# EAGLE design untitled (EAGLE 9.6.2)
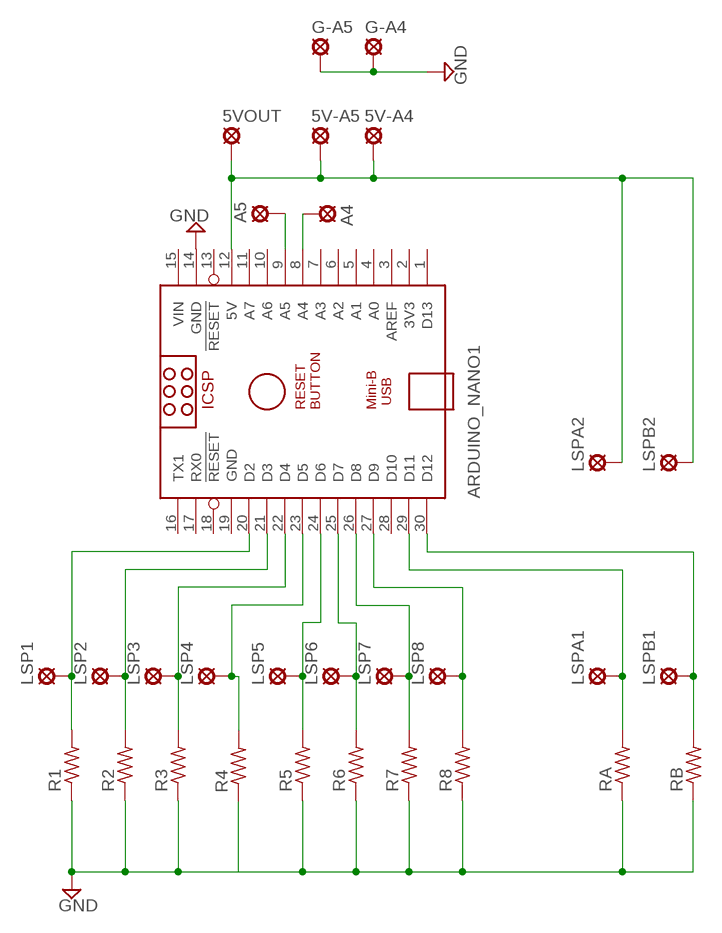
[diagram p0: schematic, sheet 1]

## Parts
5V-A4  LSP10  [LSP10]
5V-A5  LSP10  [LSP10]
5VOUT  LSP10  [LSP10]
A4  LSP10  [LSP10]
A5  LSP10  [LSP10]
ARDUINO_NANO1  ARDUINO_NANO  [ARDUINO_NANO]
G-A4  LSP10  [LSP10]
G-A5  LSP10  [LSP10]
LSP1  LSP10  [LSP10]
LSP2  LSP10  [LSP10]
LSP3  LSP10  [LSP10]
LSP4  LSP10  [LSP10]
LSP5  LSP10  [LSP10]
LSP6  LSP10  [LSP10]
LSP7  LSP10  [LSP10]
LSP8  LSP10  [LSP10]
LSPA1  LSP10  [LSP10]
LSPA2  LSP10  [LSP10]
LSPB1  LSP10  [LSP10]
LSPB2  LSP10  [LSP10]
R1  R-US_0309/12  [0309/12]
R2  R-US_0309/12  [0309/12]
R3  R-US_0309/12  [0309/12]
R4  R-US_0309/12  [0309/12]
R5  R-US_0309/12  [0309/12]
R6  R-US_0309/12  [0309/12]
R7  R-US_0309/12  [0309/12]
R8  R-US_0309/12  [0309/12]
RA  R-US_0309/12  [0309/12]
RB  R-US_0309/12  [0309/12]

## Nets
GND: ARDUINO_NANO1.14(GND) G-A4.MP G-A5.MP R1.1 R2.1 R3.1 R4.1 R5.1 R6.1 R7.1 R8.1 RA.1 RB.1
N$1: 5V-A4.MP 5V-A5.MP 5VOUT.MP ARDUINO_NANO1.12(5V) LSPA2.MP LSPB2.MP
N$2: ARDUINO_NANO1.20(D2) LSP1.MP R1.2
N$3: A5.MP ARDUINO_NANO1.9(A5)
N$4: ARDUINO_NANO1.21(D3) LSP2.MP R2.2
N$5: ARDUINO_NANO1.22(D4) LSP3.MP R3.2
N$6: ARDUINO_NANO1.23(D5) LSP4.MP R4.2
N$7: ARDUINO_NANO1.24(D6) LSP5.MP R5.2
N$8: ARDUINO_NANO1.25(D7) LSP6.MP R6.2
N$9: ARDUINO_NANO1.26(D8) LSP7.MP R7.2
N$10: ARDUINO_NANO1.27(D9) LSP8.MP R8.2
N$11: ARDUINO_NANO1.30(D12) LSPB1.MP RB.2
N$12: ARDUINO_NANO1.29(D11) LSPA1.MP RA.2
N$13: A4.MP ARDUINO_NANO1.8(A4)
Unconnected: ARDUINO_NANO1.1(D13) ARDUINO_NANO1.2(3V3) ARDUINO_NANO1.3(AREF) ARDUINO_NANO1.4(A0) ARDUINO_NANO1.5(A1) ARDUINO_NANO1.6(A2) ARDUINO_NANO1.7(A3) ARDUINO_NANO1.10(A6) ARDUINO_NANO1.11(A7) ARDUINO_NANO1.13(!RESET) ARDUINO_NANO1.16(TX1) ARDUINO_NANO1.17(RX0) ARDUINO_NANO1.18(!RESET) ARDUINO_NANO1.28(D10)

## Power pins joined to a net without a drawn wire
GND: ARDUINO_NANO1.19(GND)
VIN: ARDUINO_NANO1.15(VIN)

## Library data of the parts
5V-A4 5V-A5 5VOUT A4 A5 G-A4 G-A5 LSP1-LSP8 LSPA1 LSPA2 LSPB1 LSPB2 = solpad:LSP10: SOLDER PAD
ARDUINO_NANO1 = ArduinoNanoV30:ARDUINO_NANO: Arduino Nano V3.0 Overview: The Arduino Nano is a small, complete, and breadboard-friendly board based on the ATmega328 (Arduino Nano 3.x) or ATmega168 (Arduino Nano 2.x). It has more or less the same functionality of the Arduino Duemilanove, but in a different package. It lacks only a DC power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
R1-R8 RA RB = rcl:R-US_: RESISTOR, American symbol; SPICEPREFIX: R

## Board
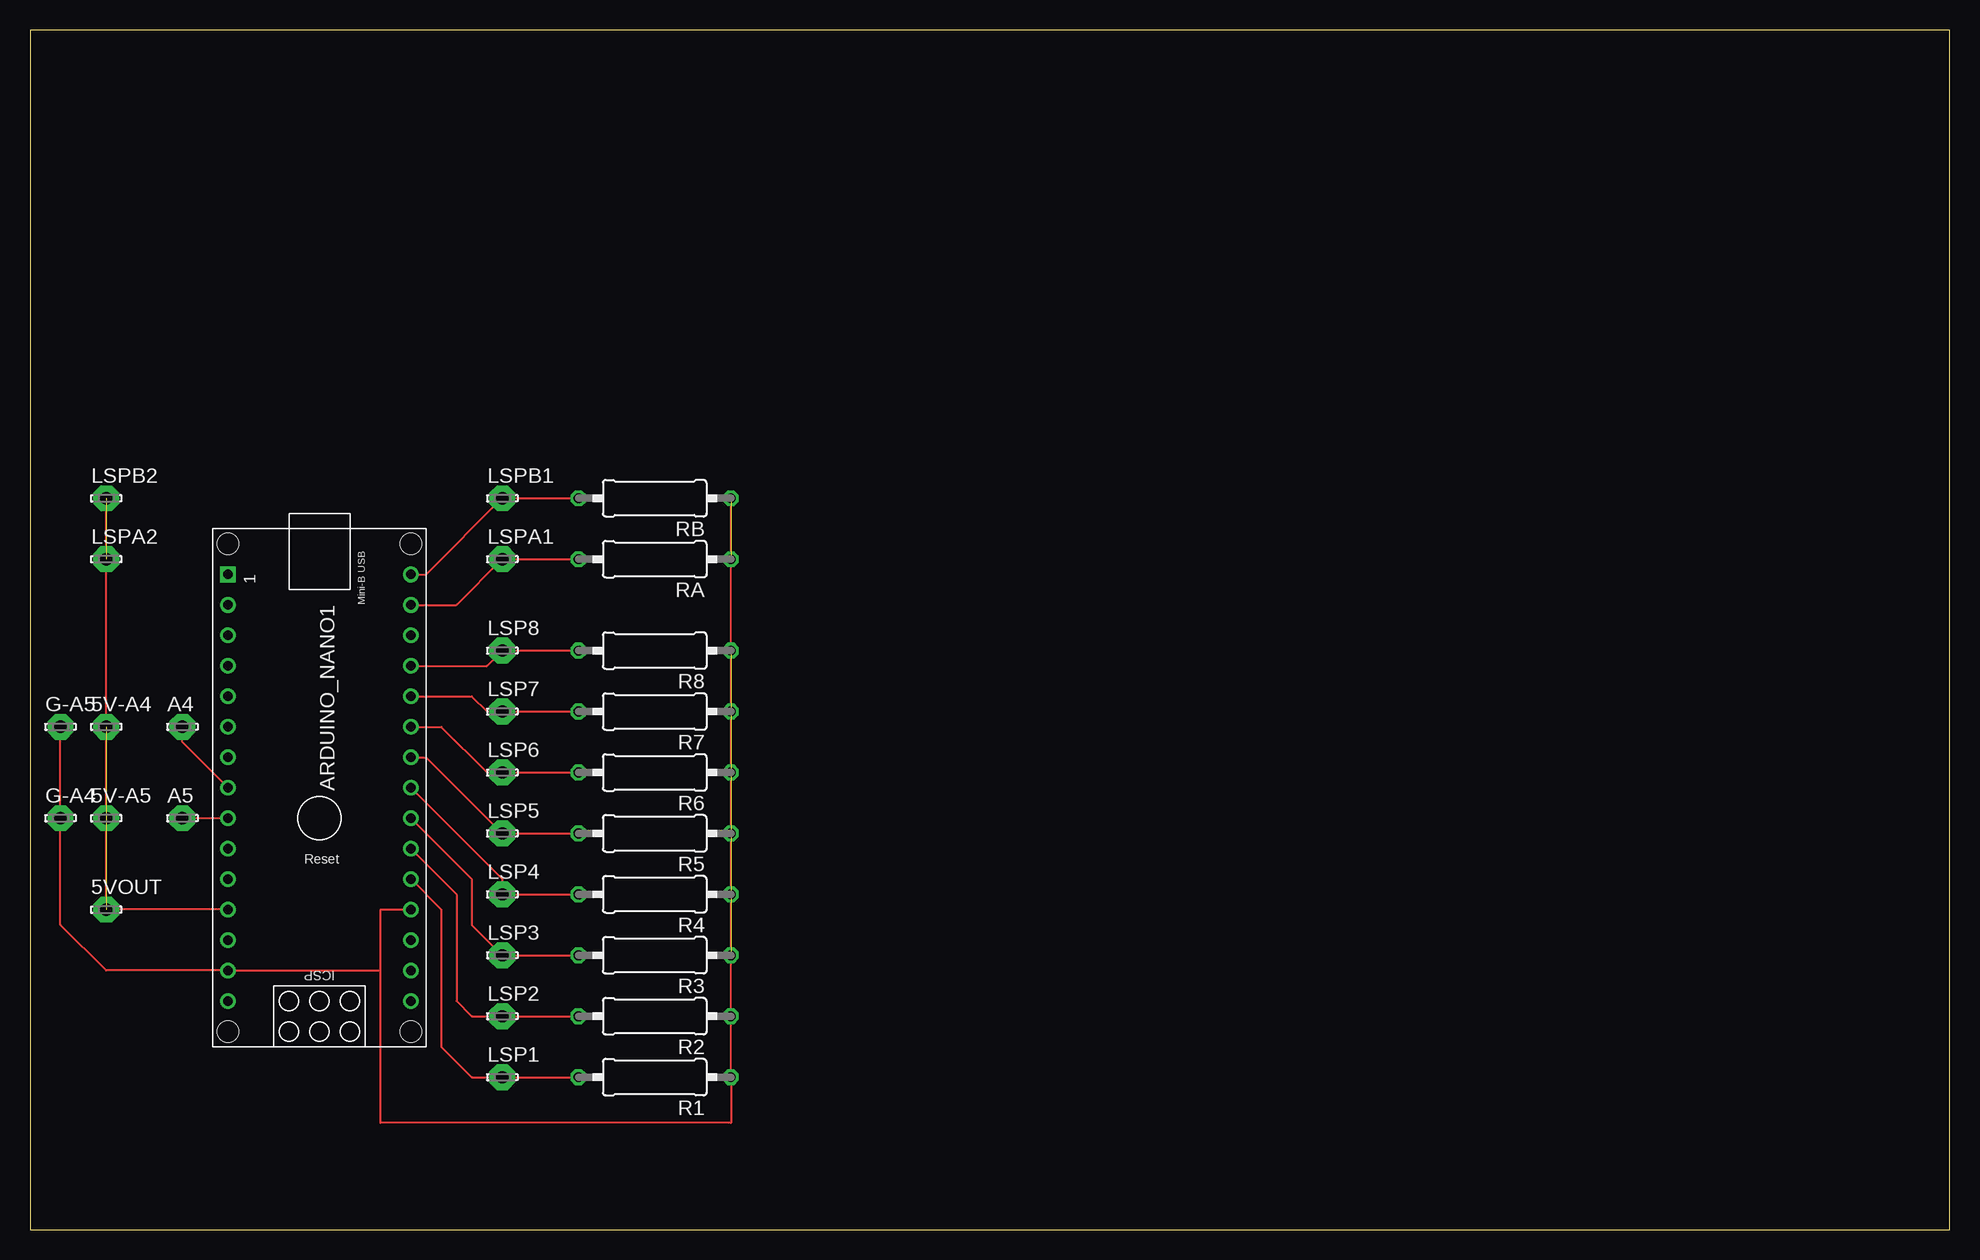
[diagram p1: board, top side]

Size 160 x 100 mm. Coordinates in mm from the lower left corner, seen from the top.
Outline: 0,0 160,0 160,100 0,100 0,0
Copper layers (1*16): Top 0.035mm / dielectric 1.5mm / Bottom 0.035mm
Design rules "default": minimum track width 6mil, minimum drill 0.35mm, track to track 6mil, track to pad 6mil, pad to pad 6mil, via to via 6mil, smd to smd 6mil, copper to edge 40mil, drill to drill 6mil, minimum pad ring 10mil, minimum via ring 8mil, stop-mask expansion 4mil, vias tented up to drill 0mil, thermal gap 10mil

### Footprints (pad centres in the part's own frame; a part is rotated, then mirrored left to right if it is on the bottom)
LSP10 = drill 1.016 pad 2.159 octagon: MP 0,0
ARDUINO_NANO = drill 0.8 square: 1 -20.32,-7.62 | drill 0.8: 2 -17.78,-7.62; 3 -15.24,-7.62; 4 -12.7,-7.62; 5 -10.16,-7.62; 6 -7.62,-7.62; 7 -5.08,-7.62; 8 -2.54,-7.62; 9 0,-7.62; 10 2.54,-7.62; 11 5.08,-7.62; 12 7.62,-7.62; 13 10.16,-7.62; 14 12.7,-7.62; 15 15.24,-7.62; 16 15.24,7.62; 17 12.7,7.62; 18 10.16,7.62; 19 7.62,7.62; 20 5.08,7.62; 21 2.54,7.62; 22 0,7.62; 23 -2.54,7.62; 24 -5.08,7.62; 25 -7.62,7.62; 26 -10.16,7.62; 27 -12.7,7.62; 28 -15.24,7.62; 29 -17.78,7.62; 30 -20.32,7.62 | hole 1.778: -22.86,-7.62; -22.86,7.62; 17.78,7.62; 17.78,-7.62
0309/12 = drill 0.813 octagon: 1 -6.35,0; 2 6.35,0

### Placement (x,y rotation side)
5V-A4  6.35,41.91 0 top
5V-A5  6.35,34.29 0 top
5VOUT  6.35,26.67 0 top
A4  12.7,41.91 0 top
A5  12.7,34.29 0 top
ARDUINO_NANO1  24.13,34.29 270 top
G-A4  2.54,34.29 0 top
G-A5  2.54,41.91 0 top
LSP1  39.37,12.7 0 top
LSP2  39.37,17.78 0 top
LSP3  39.37,22.86 0 top
LSP4  39.37,27.94 0 top
LSP5  39.37,33.02 0 top
LSP6  39.37,38.1 0 top
LSP7  39.37,43.18 0 top
LSP8  39.37,48.26 0 top
LSPA1  39.37,55.88 0 top
LSPA2  6.35,55.88 0 top
LSPB1  39.37,60.96 0 top
LSPB2  6.35,60.96 0 top
R1  52.07,12.7 180 top
R2  52.07,17.78 180 top
R3  52.07,22.86 180 top
R4  52.07,27.94 180 top
R5  52.07,33.02 180 top
R6  52.07,38.1 180 top
R7  52.07,43.18 180 top
R8  52.07,48.26 180 top
RA  52.07,55.88 180 top
RB  52.07,60.96 180 top

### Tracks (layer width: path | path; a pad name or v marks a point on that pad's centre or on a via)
GND  (6 unrouted)
  Top 0.152: RB.1 R3.1 R2.1 R1.1 58.42,8.89 29.21,8.89 29.21,21.59 | 29.21,21.59 29.21,26.67 ARDUINO_NANO1.19 | 29.21,21.59 ARDUINO_NANO1.14 6.35,21.59 2.54,25.4 G-A4.MP G-A5.MP
N$1  (3 unrouted)
  Top 0.152: ARDUINO_NANO1.12 5VOUT.MP LSPB2.MP
N$2
  Top 0.152: ARDUINO_NANO1.20 34.29,26.67 34.29,15.24 36.83,12.7 LSP1.MP R1.2
N$3
  Top 0.152: ARDUINO_NANO1.9 A5.MP
N$4
  Top 0.152: ARDUINO_NANO1.21 35.56,27.94 35.56,19.05 36.83,17.78 LSP2.MP R2.2
N$5
  Top 0.152: ARDUINO_NANO1.22 36.83,29.21 36.83,25.4 LSP3.MP R3.2
N$6
  Top 0.152: ARDUINO_NANO1.23 39.37,29.21 LSP4.MP R4.2
N$7
  Top 0.152: ARDUINO_NANO1.24 33.02,39.37 LSP5.MP R5.2
N$8
  Top 0.152: ARDUINO_NANO1.25 34.29,41.91 38.1,38.1 LSP6.MP R6.2
N$9
  Top 0.152: ARDUINO_NANO1.26 36.83,44.45 38.1,43.18 LSP7.MP R7.2
N$10
  Top 0.152: ARDUINO_NANO1.27 38.1,46.99 LSP8.MP R8.2
N$11
  Top 0.152: ARDUINO_NANO1.30 33.02,54.61 LSPB1.MP RB.2
N$12
  Top 0.152: ARDUINO_NANO1.29 35.56,52.07 LSPA1.MP RA.2
N$13
  Top 0.152: ARDUINO_NANO1.8 12.7,40.64 A4.MP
